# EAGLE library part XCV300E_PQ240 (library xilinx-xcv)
xcv300e_pq240 edit this description Auto generated by make-symbol-device-package-bsdl.ulp Rev. 26 Source: xcv300e_pq240.bsd
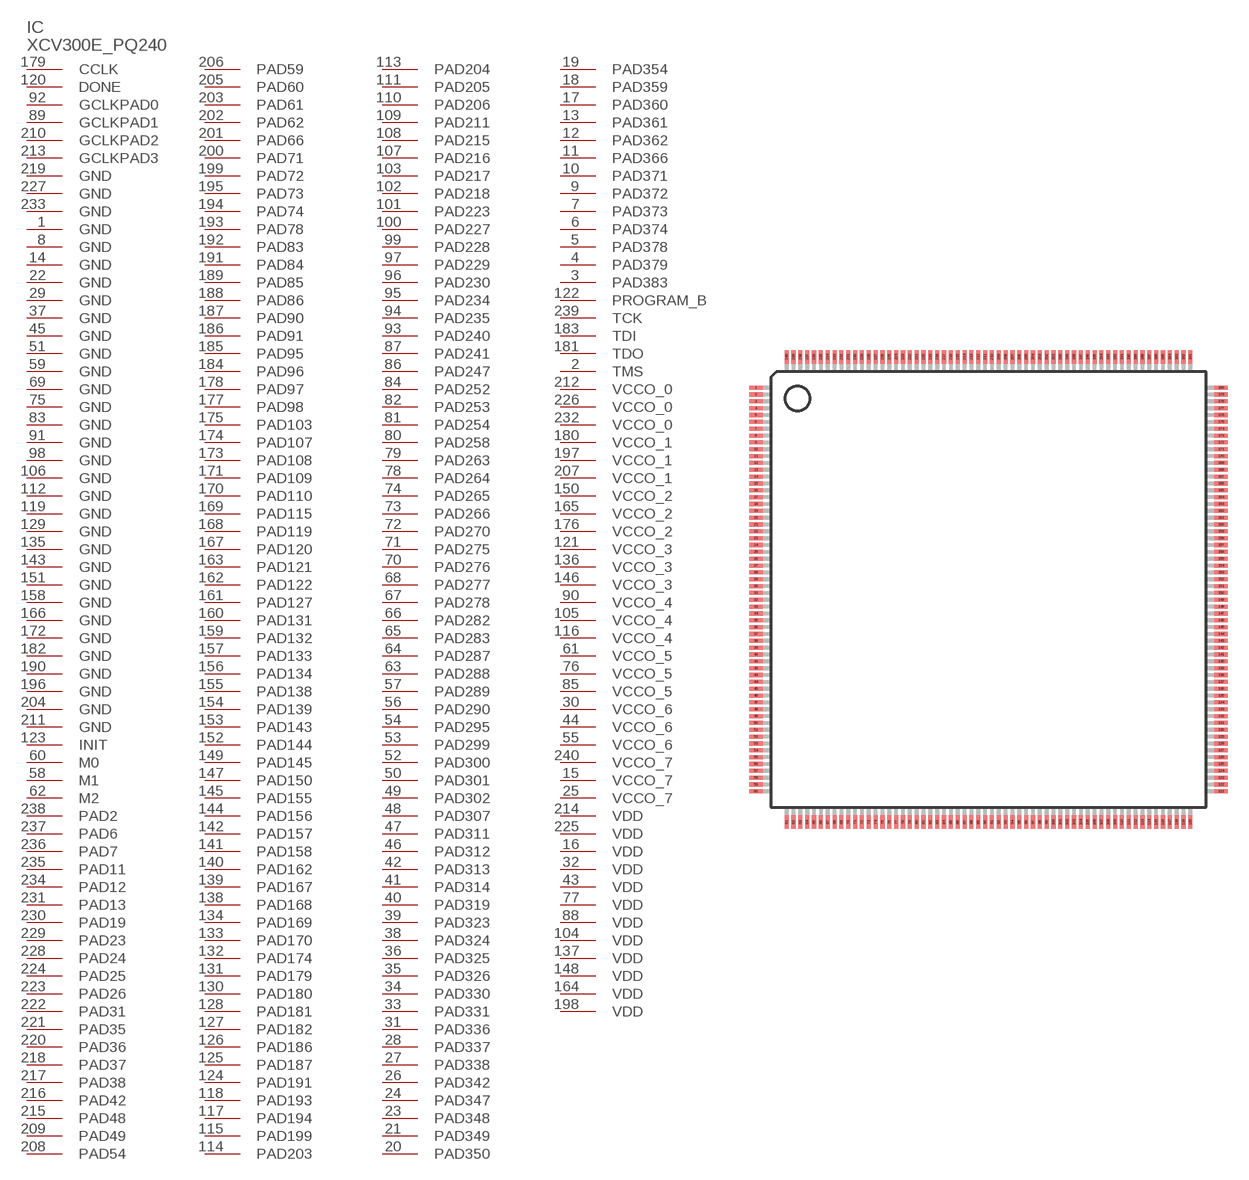
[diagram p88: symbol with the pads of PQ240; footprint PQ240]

Designator prefix IC

## XCV300E_PQ240 (OC_FARNELL: unknown; OC_NEWARK: unknown)  [PQ240]
1  GND  pwr
2  TMS  in
3  PAD383
4  PAD379
5  PAD378
6  PAD374
7  PAD373
8  GND  pwr
9  PAD372
10  PAD371
11  PAD366
12  PAD362
13  PAD361
14  GND  pwr
15  VCCO_7  pwr
16  VDD  pwr
17  PAD360
18  PAD359
19  PAD354
20  PAD350
21  PAD349
22  GND  pwr
23  PAD348
24  PAD347
25  VCCO_7  pwr
26  PAD342
27  PAD338
28  PAD337
29  GND  pwr
30  VCCO_6  pwr
31  PAD336
32  VDD  pwr
33  PAD331
34  PAD330
35  PAD326
36  PAD325
37  GND  pwr
38  PAD324
39  PAD323
40  PAD319
41  PAD314
42  PAD313
43  VDD  pwr
44  VCCO_6  pwr
45  GND  pwr
46  PAD312
47  PAD311
48  PAD307
49  PAD302
50  PAD301
51  GND  pwr
52  PAD300
53  PAD299
54  PAD295
55  VCCO_6  pwr
56  PAD290
57  PAD289
58  M1  in
59  GND  pwr
60  M0  in
61  VCCO_5  pwr
62  M2  in
63  PAD288
64  PAD287
65  PAD283
66  PAD282
67  PAD278
68  PAD277
69  GND  pwr
70  PAD276
71  PAD275
72  PAD270
73  PAD266
74  PAD265
75  GND  pwr
76  VCCO_5  pwr
77  VDD  pwr
78  PAD264
79  PAD263
80  PAD258
81  PAD254
82  PAD253
83  GND  pwr
84  PAD252
85  VCCO_5  pwr
86  PAD247
87  PAD241
88  VDD  pwr
89  GCLKPAD1  in
90  VCCO_4  pwr
91  GND  pwr
92  GCLKPAD0  in
93  PAD240
94  PAD235
95  PAD234
96  PAD230
97  PAD229
98  GND  pwr
99  PAD228
100  PAD227
101  PAD223
102  PAD218
103  PAD217
104  VDD  pwr
105  VCCO_4  pwr
106  GND  pwr
107  PAD216
108  PAD215
109  PAD211
110  PAD206
111  PAD205
112  GND  pwr
113  PAD204
114  PAD203
115  PAD199
116  VCCO_4  pwr
117  PAD194
118  PAD193
119  GND  pwr
120  DONE
121  VCCO_3  pwr
122  PROGRAM_B  in
123  INIT
124  PAD191
125  PAD187
126  PAD186
127  PAD182
128  PAD181
129  GND  pwr
130  PAD180
131  PAD179
132  PAD174
133  PAD170
134  PAD169
135  GND  pwr
136  VCCO_3  pwr
137  VDD  pwr
138  PAD168
139  PAD167
140  PAD162
141  PAD158
142  PAD157
143  GND  pwr
144  PAD156
145  PAD155
146  VCCO_3  pwr
147  PAD150
148  VDD  pwr
149  PAD145
150  VCCO_2  pwr
151  GND  pwr
152  PAD144
153  PAD143
154  PAD139
155  PAD138
156  PAD134
157  PAD133
158  GND  pwr
159  PAD132
160  PAD131
161  PAD127
162  PAD122
163  PAD121
164  VDD  pwr
165  VCCO_2  pwr
166  GND  pwr
167  PAD120
168  PAD119
169  PAD115
170  PAD110
171  PAD109
172  GND  pwr
173  PAD108
174  PAD107
175  PAD103
176  VCCO_2  pwr
177  PAD98
178  PAD97
179  CCLK
180  VCCO_1  pwr
181  TDO  out
182  GND  pwr
183  TDI  in
184  PAD96
185  PAD95
186  PAD91
187  PAD90
188  PAD86
189  PAD85
190  GND  pwr
191  PAD84
192  PAD83
193  PAD78
194  PAD74
195  PAD73
196  GND  pwr
197  VCCO_1  pwr
198  VDD  pwr
199  PAD72
200  PAD71
201  PAD66
202  PAD62
203  PAD61
204  GND  pwr
205  PAD60
206  PAD59
207  VCCO_1  pwr
208  PAD54
209  PAD49
210  GCLKPAD2  in
211  GND  pwr
212  VCCO_0  pwr
213  GCLKPAD3  in
214  VDD  pwr
215  PAD48
216  PAD42
217  PAD38
218  PAD37
219  GND  pwr
220  PAD36
221  PAD35
222  PAD31
223  PAD26
224  PAD25
225  VDD  pwr
226  VCCO_0  pwr
227  GND  pwr
228  PAD24
229  PAD23
230  PAD19
231  PAD13
232  VCCO_0  pwr
233  GND  pwr
234  PAD12
235  PAD11
236  PAD7
237  PAD6
238  PAD2
239  TCK  in
240  VCCO_7  pwr

## Footprint PQ240 (pad centres in mm)
PQ240 Auto generated by make-symbol-device-package-bsdl.ulp Rev. 26
smd 1 x 0.3: 1 -17,14.75; 2 -17,14.25; 3 -17,13.75; 4 -17,13.25; 5 -17,12.75; 6 -17,12.25; 7 -17,11.75; 8 -17,11.25; 9 -17,10.75; 10 -17,10.25; 11 -17,9.75; 12 -17,9.25; 13 -17,8.75; 14 -17,8.25; 15 -17,7.75; 16 -17,7.25; 17 -17,6.75; 18 -17,6.25; 19 -17,5.75; 20 -17,5.25; 21 -17,4.75; 22 -17,4.25; 23 -17,3.75; 24 -17,3.25; 25 -17,2.75; 26 -17,2.25; 27 -17,1.75; 28 -17,1.25; 29 -17,0.75; 30 -17,0.25; 31 -17,-0.25; 32 -17,-0.75; 33 -17,-1.25; 34 -17,-1.75; 35 -17,-2.25; 36 -17,-2.75; 37 -17,-3.25; 38 -17,-3.75; 39 -17,-4.25; 40 -17,-4.75; 41 -17,-5.25; 42 -17,-5.75; 43 -17,-6.25; 44 -17,-6.75; 45 -17,-7.25; 46 -17,-7.75; 47 -17,-8.25; 48 -17,-8.75; 49 -17,-9.25; 50 -17,-9.75; 51 -17,-10.25; 52 -17,-10.75; 53 -17,-11.25; 54 -17,-11.75; 55 -17,-12.25; 56 -17,-12.75; 57 -17,-13.25; 58 -17,-13.75; 59 -17,-14.25; 60 -17,-14.75; 121 17,-14.75; 122 17,-14.25; 123 17,-13.75; 124 17,-13.25; 125 17,-12.75; 126 17,-12.25; 127 17,-11.75; 128 17,-11.25; 129 17,-10.75; 130 17,-10.25; 131 17,-9.75; 132 17,-9.25; 133 17,-8.75; 134 17,-8.25; 135 17,-7.75; 136 17,-7.25; 137 17,-6.75; 138 17,-6.25; 139 17,-5.75; 140 17,-5.25; 141 17,-4.75; 142 17,-4.25; 143 17,-3.75; 144 17,-3.25; 145 17,-2.75; 146 17,-2.25; 147 17,-1.75; 148 17,-1.25; 149 17,-0.75; 150 17,-0.25; 151 17,0.25; 152 17,0.75; 153 17,1.25; 154 17,1.75; 155 17,2.25; 156 17,2.75; 157 17,3.25; 158 17,3.75; 159 17,4.25; 160 17,4.75; 161 17,5.25; 162 17,5.75; 163 17,6.25; 164 17,6.75; 165 17,7.25; 166 17,7.75; 167 17,8.25; 168 17,8.75; 169 17,9.25; 170 17,9.75; 171 17,10.25; 172 17,10.75; 173 17,11.25; 174 17,11.75; 175 17,12.25; 176 17,12.75; 177 17,13.25; 178 17,13.75; 179 17,14.25; 180 17,14.75
smd 0.3 x 1: 61 -14.75,-17; 62 -14.25,-17; 63 -13.75,-17; 64 -13.25,-17; 65 -12.75,-17; 66 -12.25,-17; 67 -11.75,-17; 68 -11.25,-17; 69 -10.75,-17; 70 -10.25,-17; 71 -9.75,-17; 72 -9.25,-17; 73 -8.75,-17; 74 -8.25,-17; 75 -7.75,-17; 76 -7.25,-17; 77 -6.75,-17; 78 -6.25,-17; 79 -5.75,-17; 80 -5.25,-17; 81 -4.75,-17; 82 -4.25,-17; 83 -3.75,-17; 84 -3.25,-17; 85 -2.75,-17; 86 -2.25,-17; 87 -1.75,-17; 88 -1.25,-17; 89 -0.75,-17; 90 -0.25,-17; 91 0.25,-17; 92 0.75,-17; 93 1.25,-17; 94 1.75,-17; 95 2.25,-17; 96 2.75,-17; 97 3.25,-17; 98 3.75,-17; 99 4.25,-17; 100 4.75,-17; 101 5.25,-17; 102 5.75,-17; 103 6.25,-17; 104 6.75,-17; 105 7.25,-17; 106 7.75,-17; 107 8.25,-17; 108 8.75,-17; 109 9.25,-17; 110 9.75,-17; 111 10.25,-17; 112 10.75,-17; 113 11.25,-17; 114 11.75,-17; 115 12.25,-17; 116 12.75,-17; 117 13.25,-17; 118 13.75,-17; 119 14.25,-17; 120 14.75,-17; 181 14.75,17; 182 14.25,17; 183 13.75,17; 184 13.25,17; 185 12.75,17; 186 12.25,17; 187 11.75,17; 188 11.25,17; 189 10.75,17; 190 10.25,17; 191 9.75,17; 192 9.25,17; 193 8.75,17; 194 8.25,17; 195 7.75,17; 196 7.25,17; 197 6.75,17; 198 6.25,17; 199 5.75,17; 200 5.25,17; 201 4.75,17; 202 4.25,17; 203 3.75,17; 204 3.25,17; 205 2.75,17; 206 2.25,17; 207 1.75,17; 208 1.25,17; 209 0.75,17; 210 0.25,17; 211 -0.25,17; 212 -0.75,17; 213 -1.25,17; 214 -1.75,17; 215 -2.25,17; 216 -2.75,17; 217 -3.25,17; 218 -3.75,17; 219 -4.25,17; 220 -4.75,17; 221 -5.25,17; 222 -5.75,17; 223 -6.25,17; 224 -6.75,17; 225 -7.25,17; 226 -7.75,17; 227 -8.25,17; 228 -8.75,17; 229 -9.25,17; 230 -9.75,17; 231 -10.25,17; 232 -10.75,17; 233 -11.25,17; 234 -11.75,17; 235 -12.25,17; 236 -12.75,17; 237 -13.25,17; 238 -13.75,17; 239 -14.25,17; 240 -14.75,17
